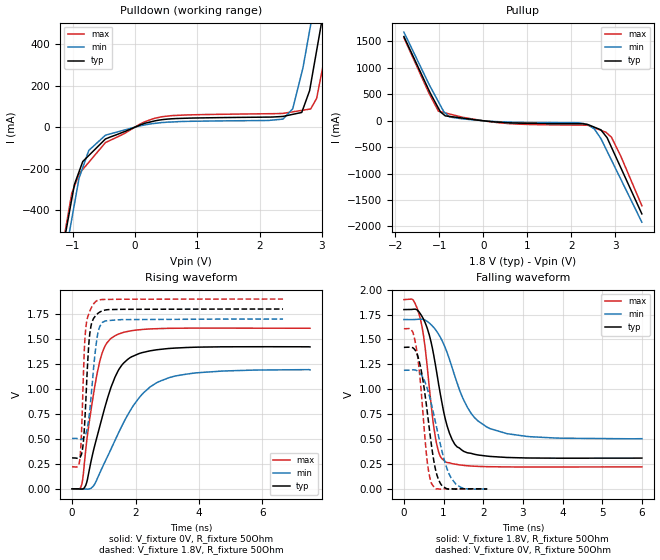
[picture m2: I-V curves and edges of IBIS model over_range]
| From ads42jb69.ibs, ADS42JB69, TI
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|   over_range Model
[Model]   over_range
Model_type   Output
Polarity   Non-Inverting
Vmeas = 0.9
Vref = 1.8
Cref = 2pF
Rref = 50
|   typ   min   max
|   (nom PVT)   (fast PVT)   (slow PVT)
 C_comp   1.903e-12   1.883e-12   1.935e-12
| Where nom  PVT is Nominal Process, 1.8V, 25C
|   Fast PVT is Strong Process,  1.9V, -40C
|   Slow PVT is Weak Process,   1.7V, 125C
[Voltage Range]   1.8   1.7   1.9
|Junction Temperature
[Temperature Range]   25   125   -40
[Pullup Reference]   1.8   1.7   1.9
[Pulldown Reference]   0   0   0
[Power Clamp Reference]   1.8   1.7   1.9
[GND Clamp Reference]   0   0   0
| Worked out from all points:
|   slope of the pulldown table from 0 to 0.27 V, typ, clamps not added: 10.2 ohm
|   slope of the pullup table from 0 to 0.27 V, typ, clamps not added: 12.7 ohm
|   falling waveform, V_fixture 1.8V, R_fixture 50Ohm: 20-80 % time 442ps typ, 731ps min, 294ps max; typ from 1.8 V to 0.31 V
|   rising waveform, V_fixture 0V, R_fixture 50Ohm: 20-80 % time 778ps typ, 1.24ns min, 472ps max; typ from 0 V to 1.42 V
|   rising waveform, V_fixture 1.8V, R_fixture 50Ohm: 20-80 % time 153ps typ, 222ps min, 123ps max; typ from 0.31 V to 1.8 V
|   falling waveform, V_fixture 0V, R_fixture 50Ohm: 20-80 % time 293ps typ, 429ps min, 215ps max; typ from 1.42 V to 0 V
[Pulldown]
|   Voltage   I(typ)   I(min)   I(max)
-1.8V     -1.78A     -1.765A    -1.815A
-1.228V   -700.6mA   -802.1mA   -689mA
-1.015V   -348mA     -444mA     -320.4mA
-741.2mV  -136.9mA   -112.3mA   -169.5mA
-472.6mV  -56.85mA   -38.62mA   -74.2mA
435.1mV   35.94mA    22.26mA    50.14mA
2.377V    51.76mA    38.85mA    66.27mA
2.531V    61.51mA    88.32mA    73.69mA
2.82V     204.7mA    492.6mA    87.53mA
2.917V    370.2mA    654.7mA    139.9mA
3.114V    707.6mA    985.4mA    441.2mA
3.6V      1.537A     1.799A     1.316A
[Pullup]
|   Voltage   I(typ)   I(min)   I(max)
-1.8V     1.593A     1.678A     1.571A
-1.227V   569.3mA    685.4mA    515.5mA
-1.016V   237.3mA    359.3mA    181.1mA
-860.4mV  92.37mA    146.1mA    148.5mA
-763.3mV  81.98mA    71.22mA    128.2mA
364.8mV   -27.52mA   -18.2mA    -38.46mA
2.151V    -56.46mA   -38.38mA   -82.4mA
2.525V    -122.2mA   -157.8mA   -133.5mA
2.669V    -171.2mA   -335.6mA   -180.3mA
2.812V    -320.7mA   -577.1mA   -238mA
2.911V    -502.1mA   -746mA     -312.3mA
3.6V      -1.762A    -1.919A    -1.607A
[Ramp]
R_load = 50
|   typ   min   max
dV/dt_r   0.852494/7.75901e-10   0.71462/1.23828e-09   0.964625/4.71475e-10
dV/dt_f   0.89414/4.40126e-10   0.717319/7.27836e-10   1.00731/2.93452e-10
[Falling Waveform]
V_fixture = 1.8V
V_fixture_min = 1.7V
V_fixture_max = 1.9V
R_fixture = 50Ohm
|   Time   V(typ)   V(min)   V(max)
0s        1.8V       1.7V       1.9V
234ps     1.803V     1.7V       1.897V
386ps     1.774V     1.703V     1.751V
534ps     1.67V      1.694V     1.424V
798ps     1.238V     1.598V     510mV
1.048ns   695.5mV    1.411V     272.8mV
1.282ns   448.8mV    1.136V     249.4mV
1.598ns   363.1mV    821.5mV    232.8mV
2.168ns   326.6mV    605.9mV    223.1mV
6ns       309.8mV    504.5mV    221.2mV
[Rising Waveform]
V_fixture = 0V
V_fixture_min = 0V
V_fixture_max = 0V
R_fixture = 50Ohm
|   Time   V(typ)   V(min)   V(max)
0s        1.005nV    49.26nV    167.8pV
308ps     -3.255mV   -412.2uV   45.01mV
462ps     64.43mV    -3.351mV   477.5mV
794ps     529.3mV    101.3mV    1.16V
1.006ns   783.2mV    249.2mV    1.407V
1.236ns   1.023V     403.5mV    1.508V
1.768ns   1.3V       747.3mV    1.577V
2.732ns   1.394V     1.073V     1.604V
3.992ns   1.419V     1.163V     1.609V
7.5ns     1.421V     1.191V     1.608V
[Rising Waveform]
V_fixture = 1.8V
V_fixture_min = 1.7V
V_fixture_max = 1.9V
R_fixture = 50Ohm
|   Time   V(typ)   V(min)   V(max)
0s        309.8mV    504.5mV    221.2mV
228ps     308.8mV    497.6mV    259mV
280ps     331.5mV    495.8mV    439.1mV
324ps     385.7mV    499.9mV    796.1mV
390ps     612.4mV    520.7mV    1.411V
440ps     920.3mV    557.4mV    1.628V
562ps     1.561V     795.5mV    1.781V
748ps     1.736V     1.418V     1.875V
1.048ns   1.791V     1.681V     1.896V
6.65ns    1.8V       1.7V       1.9V
[Falling Waveform]
V_fixture = 0V
V_fixture_min = 0V
V_fixture_max = 0V
R_fixture = 50Ohm
|   Time   V(typ)   V(min)   V(max)
0s        1.421V     1.191V     1.608V
184ps     1.423V     1.194V     1.6V
298ps     1.385V     1.192V     1.45V
392ps     1.272V     1.167V     1.173V
586ps     782.6mV    1.012V     282.2mV
704ps     411.3mV    834.3mV    49.82mV
904ps     67.9mV     474.2mV    -2.015mV
1.194ns   503.3uV    108.3mV    1.696mV
1.544ns   1.297mV    2.206mV    338uV
2.1ns     838.3pV    49.05nV    65.42pV
